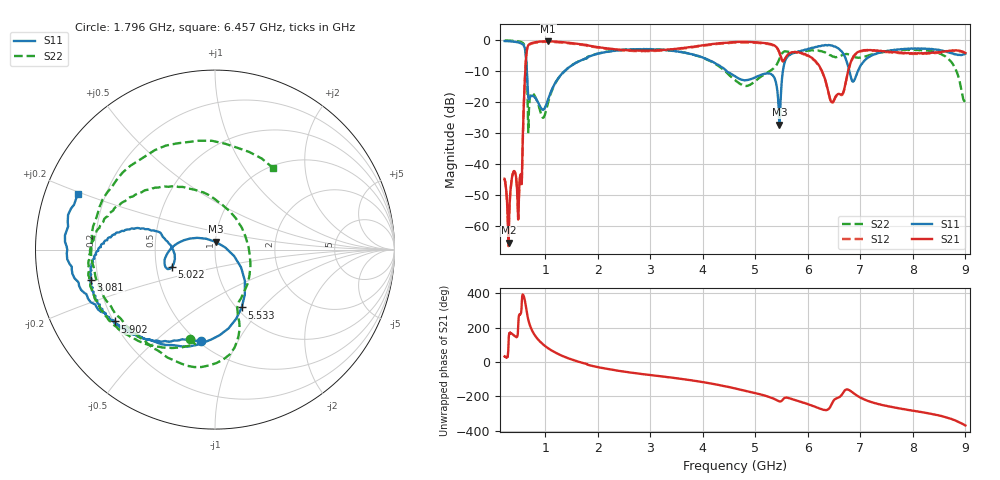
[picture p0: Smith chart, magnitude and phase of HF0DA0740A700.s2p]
!Agilent Technologies,E8358A,US41080443,A.07.50.56
!Agilent E8358A: A.07.50.56
!Date: Wednesday, May 11, 2016 14:50:26
!Correction: S11(Full 2 Port(1,2))
!S21(Full 2 Port(1,2))
!S12(Full 2 Port(1,2))
!S22(Full 2 Port(1,2))
!S2P File: Measurements: S11, S21, S12, S22:Log Frequency Sweep
# Hz S  dB  R 50
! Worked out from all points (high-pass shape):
!   1601 points, 225 MHz to 9 GHz, reference 50 ohm
!   highest |S21| = -0.31 dB at 1.057 GHz (marker M1); lowest = -65.3 dB at 299.5 MHz (marker M2)
!   |S21| within 3 dB of the highest: 647.7 MHz to 2.697 GHz (2.05 GHz wide, 123 % of centre); 3.036 GHz to 5.444 GHz (2.408 GHz wide, 56.8 % of centre)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
!   lowest |S11| = -27.2 dB at 5.457 GHz (marker M3), VSWR 1.09, Z = 50.1 + j4.38 ohm
!   |S11| at or under -10 dB: 649.3 MHz to 1.362 GHz (712.7 MHz wide, 70.9 % of centre); 4.457 GHz to 5.524 GHz (1.067 GHz wide, 21.4 % of centre); 6.792 GHz to 6.951 GHz (159.1 MHz wide, 2.32 % of centre)
!   |S22| runs from -29.6 to 0.0 dB; largest |S21 - S12| = 0.023
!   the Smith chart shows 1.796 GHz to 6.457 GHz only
!   S11 on the Smith chart (normalised r, x): 1.796 GHz: 0.51, -0.72; 3.081 GHz: 0.17, -0.12; 5.022 GHz: 0.60, -0.12; 5.533 GHz: 1.06, -0.78; 5.902 GHz: 0.21, -0.31; 6.457 GHz: 0.10, +0.19
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2.25e8  -0.23 -71.5  -44.63 33.0  -44.75 33.3  -0.05 -46.5
2.994623e8  -0.31 -96.4  -65.29 114.8  -65.46 117.9  -0.09 -63.5
3.885865e8  -0.41 -129.4  -42.56 159.0  -42.77 159.2  -0.16 -86.9
4.859734e8  -0.69 -174.4  -57.26 -133.7  -57.45 -133.2  -0.34 -119.9
5.911831e8  -1.74 101.5  -20.51 22.3  -20.67 22.4  -1.25 174.7
6.558128e8  -12.25 2.8  -2.54 -84.0  -2.71 -83.9  -14.41 65.7
7.635982e8  -17.95 -27.1  -0.78 174.8  -0.95 175.0  -17.13 -162.0
1.05693e9  -18.87 -48.5  -0.31 79.9  -0.49 80.1  -19.80 18.1
1.687749e9  -6.39 -92.8  -1.28 -2.6  -1.45 -2.5  -6.38 -94.2
1.79615e9  -5.73 -98.7  -1.51 -11.5  -1.68 -11.4  -5.74 -105.7
3.08066e9  -2.95 -166.4  -3.27 -78.5  -3.45 -78.3  -2.92 -170.0
3.152512e9  -3.02 -168.4  -3.22 -80.9  -3.40 -80.7  -2.99 -172.7
4.622431e9  -11.71 172.4  -0.54 -153.3  -0.72 -153.3  -12.93 66.4
5.022463e9  -11.74 -158.2  -0.64 178.0  -0.83 178.1  -12.85 -31.5
5.457115e9  -27.19 86.0  -3.84 131.5  -4.03 131.5  -6.06 -74.7
5.53313e9  -8.99 -65.2  -6.68 145.3  -6.87 145.6  -3.80 -92.9
5.902105e9  -3.28 -144.3  -4.23 124.7  -4.41 124.9  -3.61 -151.3
6.081681e9  -2.40 -158.9  -5.71 106.4  -5.90 106.4  -3.23 -179.7
6.457391e9  -1.67 158.0  -20.01 118.3  -20.23 118.1  -5.07 54.7
6.840523e9  -13.04 1.8  -6.10 -174.0  -6.31 -173.5  -5.06 -113.0
7.553438e9  -3.37 -162.2  -3.73 102.0  -3.88 102.0  -3.56 -176.1
9e9  -4.32 -170.3  -4.09 -8.5  -4.23 -8.7  -18.27 -69.8
